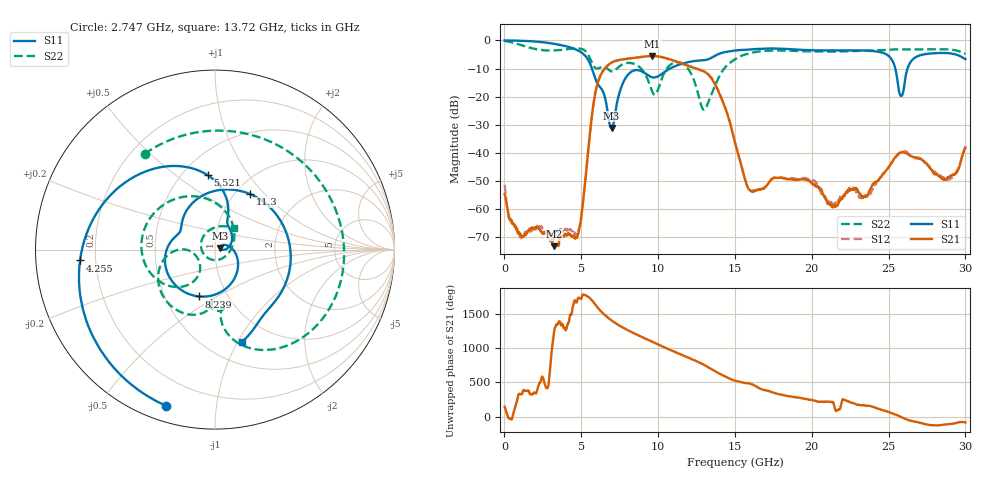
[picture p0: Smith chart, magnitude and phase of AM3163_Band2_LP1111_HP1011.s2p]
!Agilent Technologies,E8364B,MY43040894,A.07.50.67
!Agilent E8364B: A.07.50.67
!Date: Thursday, August 20, 2020 12:09:27
!Correction: S11(Full 2 Port(1,2))
!S21(Full 2 Port(1,2))
!S12(Full 2 Port(1,2))
!S22(Full 2 Port(1,2))
!S2P File: Measurements: S11, S21, S12, S22:
# Hz S  dB  R 50
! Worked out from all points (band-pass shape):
!   3201 points, 10 MHz to 30 GHz, reference 50 ohm
!   highest |S21| = -5.56 dB at 9.626 GHz (marker M1); lowest = -73.2 dB at 3.234 GHz (marker M2)
!   |S21| within 3 dB of the highest: 6.788 GHz to 11.74 GHz (4.948 GHz wide, 53.4 % of centre)
!   lowest |S11| = -31.1 dB at 6.973 GHz (marker M3), VSWR 1.06, Z = 52.7 + j0.88 ohm
!   |S11| at or under -10 dB: 5.694 GHz to 10.78 GHz (5.084 GHz wide, 61.7 % of centre); 25.44 GHz to 26.23 GHz (794.8 MHz wide, 3.08 % of centre)
!   |S22| runs from -24.7 to -0.2 dB; largest |S21 - S12| = 0.012
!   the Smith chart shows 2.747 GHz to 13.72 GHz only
!   S11 on the Smith chart (normalised r, x): 2.747 GHz: 0.07, -0.73; 4.255 GHz: 0.14, -0.04; 5.521 GHz: 0.66, +0.66; 8.239 GHz: 0.74, -0.42; 11.3 GHz: 1.16, +0.83; 13.72 GHz: 0.72, -1.04
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1e7  -0.01 -2.7  -54.67 143.8  -51.37 -12.1  -0.17 -6.7
1.003419e9  -0.10 -38.5  -69.05 -33.8  -69.53 149.5  -1.50 -94.1
2.746588e9  -0.80 -107.4  -68.27 52.3  -69.43 -61.8  -3.58 126.3
3.233925e9  -1.19 -127.8  -73.20 164.1  -70.35 -1.6  -3.57 90.8
4.255459e9  -2.45 -175.4  -69.17 24.3  -67.14 -113.3  -3.01 19.0
5.014581e9  -4.32 138.5  -62.36 -76.7  -61.47 -25.5  -3.02 -37.3
5.520662e9  -7.63 95.4  -35.27 -66.4  -35.39 -67.2  -5.88 -78.8
6.973303e9  -31.13 17.5  -7.86 -39.3  -7.90 -39.3  -11.00 -95.6
8.238506e9  -11.19 -108.7  -6.33 154.5  -6.36 154.9  -8.05 -131.6
9.625544e9  -13.12 155.6  -5.56 8.7  -5.55 8.6  -18.32 -170.1
1.000979e10  -12.73 144.0  -5.70 -31.0  -5.72 -31.3  -17.28 -127.2
1.130311e10  -8.73 57.9  -7.71 -158.3  -7.91 -157.3  -7.72 167.5
1.372105e10  -5.42 -73.8  -15.81 -61.8  -15.54 -60.8  -15.92 47.5
1.5005e10  -3.58 -131.7  -36.33 161.6  -36.31 160.6  -6.70 -112.3
1.599842e10  -3.22 -173.3  -53.40 118.0  -53.50 120.5  -4.52 -172.2
1.787279e10  -2.91 98.3  -48.89 -35.0  -48.79 -34.9  -3.57 91.9
2.000958e10  -3.50 -10.0  -50.83 -118.4  -49.90 -122.1  -3.93 -9.5
2.231506e10  -3.54 -100.0  -53.42 -137.3  -54.21 -146.6  -3.86 -93.9
2.500479e10  -5.52 157.8  -45.16 64.5  -44.88 67.3  -3.36 -167.9
2.582014e10  -19.76 171.9  -39.84 -8.2  -39.71 -7.4  -3.21 170.0
2.728216e10  -4.97 156.7  -43.05 -105.3  -42.72 -104.4  -3.18 132.4
3e10  -6.67 52.1  -38.26 -87.0  -37.62 -86.9  -4.76 55.1
